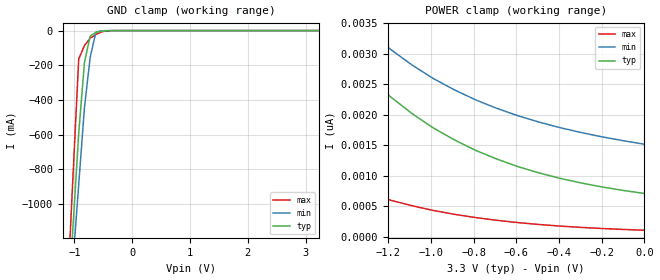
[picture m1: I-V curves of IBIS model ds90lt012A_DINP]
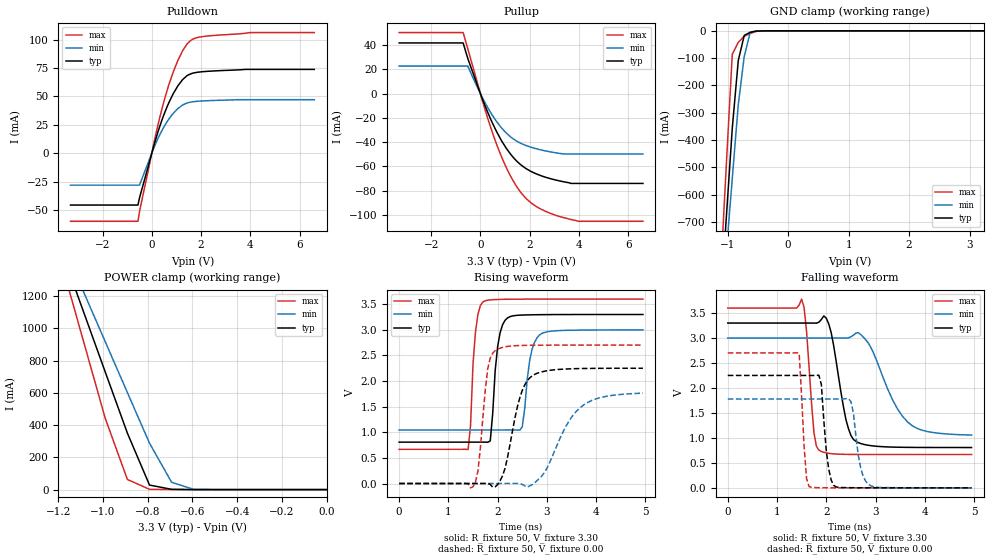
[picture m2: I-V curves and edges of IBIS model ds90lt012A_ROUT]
|   National Semiconductor Corporation
|   IBIS Model of DS90LT012A
|   3V LVDS Single CMOS Differential Line Receiver
|   8 Lead LLP Package
[IBIS Ver]   3.2
[Comment Char]   |_char
[File name]   ds90lt012atld.ibs
[File Rev]   1.0
[Date]   5/25/07
[Source]
SPICE to IBIS Translation
[Notes]
* Rev 1.0 Comments:
Parser Results:
Checking ds90lt012atld.ibs for IBIS 3.2 Compatibility...
Errors  : 0
File Passed
Model Comments:
Created By: dglisic
* END Rev 1.0 Comments
[Disclaimer]
(C) Copyright National Semiconductor Corporation 2002
   All rights reserved
   National Semiconductor Corporation hereby grants
the user of this IBIS model a non-exclusive, nontransferable
license to use this IBIS model under the following terms.
Before using this IBIS model, the user should read this
license.  If the user does not accept these terms,  the
IBIS model should be returned to National within 30 days.
   The user is granted this license only to use the
IBIS model and is not granted rights to sell, load, rent,
lease or license the IBIS model in whole or in part, or in
modified form to anyone other than user. User may modify
the IBIS model to suit its specific applications but rights
to derivative works and such modifications shall belong to
National.
   This IBIS model is provided on an "AS IS" basis and
National makes absolutely no warranty with respect to the
information contained herein.NATIONAL DISCLAIMS AND CUSTOMER
WAIVES ALL WARRANTIES, EXPRESS OR IMPLIED, INCLUDING
WARRANTIES OF MERCHANTABILITY OR FITNESS FOR A PARTICULAR
PURPOSE. The entire risk as to quality and performance is
with the Customer. ACCORDINGLY, IN NO EVENT SHALL THE
COMPANY BE LIABLE FOR ANY DAMAGES, WHETHER IN CONTRACT OR
TORT,INCLUDING ANY LOST PROFITS OR OTHER INCIDENTAL,
CONSEQUENTIAL, EXEMPLARY, OR PUNITIVE DAMAGES ARISING OUT
OF THE USE OR APPLICATION OF THE IBIS model provided in
this package.Further, National reserves the right to make
changes without notice to any product herein to improve
reliability, function, or design. National does not convey
any license under patent rights or any other intellectual
property rights, including those of third parties.
   National is not obligated to provide maintenance or support
for the licensed IBIS model.
Contact National at ATTN:INTERFACE APPLICATIONS/IBIS MODELS.
5 Foden Road, M/S 03-03, South Porltand, ME 04106
(207) 541-6031
[Copyright]
(c) Copyright 2002 National Semiconductor Corp.
[Component]   DS90LT012A
Si_location Pin
Timing_location Pin
[Manufacturer]   National Semiconductor Corp.
[Package]
|   TYP   MIN   MAX
R_pkg   1.000m   1.000m   1.000m
L_pkg   0.008n   0.008n   0.008n
C_pkg   0.030p   0.030p   0.030p
[Pin]   signal_name   model_name   R_pin   L_pin   C_pin
1   in-   ds90lt012A_DINM   1.000m  0.008n  0.030p
2   gnd   GND   1.000m  0.008n  0.030p
3   in+   ds90lt012A_DINP   1.000m  0.008n  0.030p
4   nc   NC   1.000m  0.008n  0.030p
5   nc   NC   1.000m  0.008n  0.030p
6   vdd   POWER   1.000m  0.008n  0.030p
7   gnd   GND   1.000m  0.008n  0.030p
8   ttl_out   ds90lt012A_ROUT   1.000m  0.008n  0.030p
[Series Pin Mapping]   pin_2   model_name
3   1   term_resistor
[Diff Pin] inv_pin   vdiff   tdelay_typ   tdelay_min   tdelay_max
| The '+' pin is Diff_pin and the '-' pin is the inv_pin
| Receiver Vth = +/-30mV
3   1   30mv   0   0   0
|   Model resistor
[Model]   term_resistor
Model_type   Series
Polarity   Non-Inverting
C_comp   0.0pF   0.0pF   0.0pF
[Temperature Range] 25   85   -40
[Voltage Range]   3.300   3.0   3.6
| Resistance   ohm(typ)   ohm(min)   ohm(max)
[R Series]   100   85   115
| Models and submodels in the file (4): ds90lt012A_DINP (Input), ds90lt012A_DINM (Input), ds90lt012A_ROUT (3-state), term_resistor (Series)
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[Model]   ds90lt012A_DINP
Model_type Input
Vinh=.030
Vinl=-.030
|   TYP   MIN   MAX
C_comp   3p   3p   3p
[Temperature Range] 25   85   -40
[Voltage Range]   3.30   3.00   3.60
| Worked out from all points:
|   GND clamp passes 1 mA (typ) near -0.44 V on its own axis
[GND Clamp]
|V(groundclamp)   I(typ)   I(min)   I(max)
-3.3V     -13.99A    -11.84A    -17.64A
-1.122V   -1.67A     -1.778A    -1.527A
-1.023V   -1.13A     -1.332A    -837.2mA
-924mV    -590.9mA   -886.9mA   -163.5mA
-825mV    -184.1mA   -443.9mA   -85.98mA
-726mV    -31.28mA   -154mA     -44.22mA
-627mV    -11.3mA    -9.067mA   -22.94mA
-528mV    -2.884mA   -1.121mA   -6.911mA
-330mV    -102.9uA   -43.73uA   -230uA
3.234V    680.1pA    1.665nA    71.95pA
[POWER Clamp]
|V(table)   I(typ)   I(min)   I(max)
-3.267V   37.11nA    32.01nA    15.98nA
-2.277V   10.28nA    10.18nA    3.62nA
-2.178V   8.962nA    9.038nA    3.088nA
-1.98V    6.807nA    7.149nA    2.241nA
-1.881V   5.933nA    6.374nA    1.908nA
-1.683V   4.498nA    5.089nA    1.374nA
-1.485V   3.419nA    4.109nA    986.4pA
-1.287V   2.615nA    3.371nA    707.3pA
-1.089V   2.023nA    2.82nA     508.3pA
-891mV    1.591nA    2.412nA    367.6pA
-495mV    1.048nA    1.882nA    200pA
0V        708.6pA    1.517nA    105.1pA
[Model]   ds90lt012A_ROUT
Model_type 3-state
Enable Active-High
Polarity Non-Inverting
Vref=0.00
Vmeas=1.65
Rref=500
Cref=15p
| Cref of 15pF is total jig capacitance (distributed)
|   TYP   MIN   MAX
C_comp   4p   4p   4p
[Temperature Range] 25   85   -40
[Voltage Range]   3.30   3.00   3.60
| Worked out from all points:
|   slope of the pulldown table from 0 to 0.495 V, typ, clamps not added: 14.5 ohm
|   slope of the pullup table from 0 to 0.495 V, typ, clamps not added: 20.2 ohm
|   GND clamp passes 1 mA (typ) near -0.51 V on its own axis
|   POWER clamp passes 1 mA (typ) near -0.65 V on its own axis
|   falling waveform, R_fixture 50, V_fixture 3.30: 20-80 % time 258ps typ, 543ps min, 129ps max; typ from 3.3 V to 0.808 V
|   falling waveform, R_fixture 50, V_fixture 0.00: 20-80 % time 121ps typ, 153ps min, 92ps max; typ from 2.25 V to 0 V
|   rising waveform, R_fixture 50, V_fixture 3.30: 20-80 % time 130ps typ, 151ps min, 103ps max; typ from 0.808 V to 3.3 V
|   rising waveform, R_fixture 50, V_fixture 0.00: 20-80 % time 307ps typ, 572ps min, 157ps max; typ from 0 V to 2.25 V
[Pullup]
|Vtable   I(typ)   I(min)   I(max)
-3.3V     41.78mA    22.7mA     50.33mA
-700mV    41.78mA    22.7mA     50.33mA
-512mV    29.03mA    22.7mA     36.91mA
300mV     -15.55mA   -11.59mA   -20.51mA
862mV     -38.95mA   -28.35mA   -52.32mA
1.425V    -54.59mA   -38.51mA   -75.06mA
1.675V    -59.21mA   -41.24mA   -82.3mA
2.05V     -64.06mA   -44.15mA   -89.91mA
2.862V    -70.17mA   -48.06mA   -98.81mA
3.675V    -73.99mA   -49.71mA   -103.7mA
3.987V    -73.99mA   -49.71mA   -105.2mA
6.6V      -73.99mA   -49.71mA   -105.2mA
[Pulldown]
|V(pulldown)   I(typ)   I(min)   I(max)
-3.3V     -45.6mA    -28.09mA   -59.93mA
-562.5mV  -45.6mA    -28.09mA   -59.93mA
-500mV    -39.41mA   -28.09mA   -51.57mA
250mV     18.81mA    12.97mA    24.97mA
625mV     41.14mA    27.9mA     55.5mA
875mV     52.59mA    35.22mA    71.76mA
1.062V    59.45mA    39.4mA     81.87mA
1.438V    68.45mA    44.3mA     96.41mA
1.625V    70.29mA    45.22mA    99.98mA
2.188V    72.04mA    46.22mA    103.1mA
4V        73.87mA    47.18mA    106.3mA
6.6V      73.87mA    47.18mA    106.3mA
[GND Clamp]
|V(groundclamp)   I(typ)   I(min)   I(max)
-3.3V     -8.298A    -7.144A    -10.19A
-1.122V   -1.014A    -1.085A    -910.4mA
-1.023V   -685.2mA   -813mA     -493.8mA
-924mV    -356.9mA   -541.1mA   -86.03mA
-825mV    -109.1mA   -270.4mA   -42.2mA
-726mV    -16.67mA   -93.38mA   -19.78mA
-627mV    -5.397mA   -5.071mA   -9.53mA
-528mV    -1.147mA   -525.3uA   -2.217mA
-330mV    -29.9uA    -17uA      -40.54uA
3.234V    800.7pA    480.8nA    91.27pA
[POWER Clamp]
|V(table)   I(typ)   I(min)   I(max)
-3.267V   9.584A     8.291A     11.75A
-1.188V   1.491A     1.55A      1.416A
-1.089V   1.11A      1.233A     928.2mA
-990mV    729.5mA    917.3mA    441.9mA
-891mV    350.5mA    602.3mA    63.05mA
-792mV    28.24mA    288.1mA    1.817mA
-693mV    1.617mA    45.27mA    453.5uA
-594mV    118.9uA    1.221mA    66.77uA
0V        857.1pA    1.83nA     132.3pA
[Ramp]
|   TYP   MIN   MAX
dV/dt_r   1.496V/0.258ns   1.160V/0.540ns   1.758V/0.127ns
dV/dt_f   1.349V/0.305ns   1.059V/0.586ns   1.620V/0.152ns
R_load=50
[Falling Waveform]
R_fixture=50
V_fixture=3.30
V_fixture_min=3.00
V_fixture_max=3.60
|Time   V(typ)   V(min)   V(max)
0s        3.3V       3V         3.6V
1.5ns     3.3V       3V         3.779V
1.6ns     3.3V       3V         3.13V
1.75ns    3.299V     3V         1.105V
1.85ns    3.317V     3V         757.3mV
2.05ns    3.283V     3V         691mV
2.55ns    971.2mV    3.056V     669.1mV
2.85ns    853.4mV    2.905V     668mV
3.65ns    811mV      1.32V      667.7mV
4.95ns    807.8mV    1.057V     667.7mV
[Falling Waveform]
R_fixture=50
V_fixture=0.00
V_fixture_min=0.00
V_fixture_max=0.00
|Time   V(typ)   V(min)   V(max)
0s        2.251V     1.779V     2.702V
1.45ns    2.251V     1.779V     2.692V
1.55ns    2.251V     1.779V     830.9mV
1.65ns    2.251V     1.779V     26.87mV
1.9ns     2.071V     1.779V     2.863mV
2ns       746.2mV    1.779V     1.697mV
2.15ns    50.12mV    1.779V     783.1uV
2.5ns     3.28mV     1.728V     174.4uV
2.9ns     911.4uV    43.52mV    55.09uV
4.95ns    21.66uV    183uV      1.585uV
[Rising Waveform]
R_fixture=50
V_fixture=3.30
V_fixture_min=3.00
V_fixture_max=3.60
|Time   V(typ)   V(min)   V(max)
0s        807.7mV    1.045V     667.7mV
1.4ns     807.7mV    1.045V     662.6mV
1.55ns    807.7mV    1.045V     2.96V
1.7ns     807.8mV    1.045V     3.544V
1.85ns    831.5mV    1.045V     3.585V
2ns       2.675V     1.045V     3.593V
2.2ns     3.232V     1.046V     3.598V
2.5ns     3.289V     1.108V     3.599V
2.85ns    3.296V     2.9V       3.6V
4.95ns    3.3V       3V         3.6V
[Rising Waveform]
R_fixture=50
V_fixture=0.00
V_fixture_min=0.00
V_fixture_max=0.00
|Time   V(typ)   V(min)   V(max)
0s        2.096nV    24.16nV    108.1pV
1.5ns     20.18nV    21.62nV    -62.51mV
1.6ns     72.45nV    24.1nV     244.3mV
1.8ns     839.7uV    23.79nV    2.245V
2ns       -21.01mV   716.9nV    2.623V
2.15ns    295.4mV    -11.38uV   2.668V
2.45ns    1.674V     -1.813mV   2.695V
2.7ns     2.102V     -23.23mV   2.7V
3.7ns     2.245V     1.5V       2.702V
4.95ns    2.25V      1.763V     2.702V
